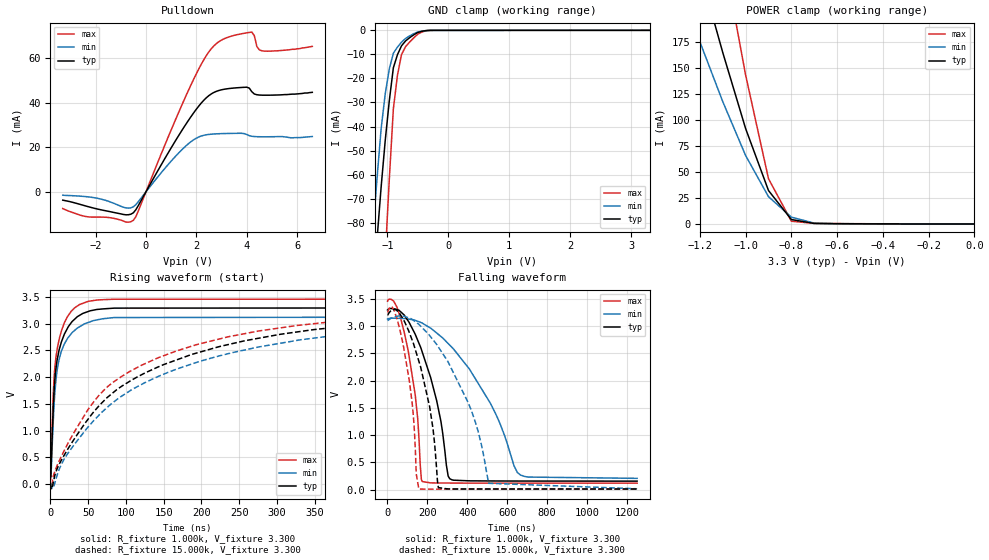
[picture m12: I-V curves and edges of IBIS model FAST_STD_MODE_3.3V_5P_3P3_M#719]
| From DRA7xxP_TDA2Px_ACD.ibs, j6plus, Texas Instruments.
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| Model based on original model for BI2C1833DVFZP18_SSCEV
|   Sub model FAST_STD_MODE_3.3V_5P_3P3
[model]   FAST_STD_MODE_3.3V_5P_3P3_M#719
|[Description]  [3.3V-I/O_OPEN_DRAIN-X-FAST MODE AND STD MODE, IND, 5 PERCENT%]
|   FAST MODE AND STD MODE, ,IND,5 PERCENT%
|[Input Load]
|[Output Drive] FAST MODE AND STD MODE
|Voltage   3.3V
|Mode   I/O_OPEN_DRAIN
Model_type   I/O_open_drain
Polarity   Non-Inverting
Enable   Active-Low
Vinl =  0.99
Vinh =  2.31
Cref =  15pF
Rref =  1000
Vref =  3.3V
Vmeas =  1.65
C_comp   2.155p   1.84p   2.47p
[Model Spec]
Vinl   0.99   0.9405   1.0395
Vinh   2.31   2.1945   2.4255
[Temperature Range]   25   125   -40
[Voltage Range]   3.3   3.135   3.465
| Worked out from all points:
|   slope of the pulldown table from 0 to 0.495 V, typ, clamps not added: 49.9 ohm
|   GND clamp passes 1 mA (typ) near -0.51 V on its own axis
|   POWER clamp passes 1 mA (typ) near -0.71 V on its own axis
|   rising waveform, R_fixture 1.000k, V_fixture 3.300: 20-80 % time 12.7ns typ, 13.7ns min, 11.4ns max; typ from 0.154 V to 3.3 V
|   rising waveform, R_fixture 15.000k, V_fixture 3.300: 20-80 % time 199ns typ, 223ns min, 173ns max; typ from 0.011 V to 3.2 V
|   falling waveform, R_fixture 1.000k, V_fixture 3.300: 20-80 % time 125ns typ, 266ns min, 69.9ns max; typ from 3.3 V to 0.155 V
|   falling waveform, R_fixture 15.000k, V_fixture 3.300: 20-80 % time 101ns typ, 203ns min, 58.8ns max; typ from 3.2 V to 0.011 V
[POWER_clamp]
-3.3V     2.049A     1.823A     3.216A
-1.233V   270.7mA    195.6mA    431mA
-1.2V     243.7mA    175.4mA    388.1mA
-1.133V   191.3mA    137mA      304.3mA
-1.1V     165.1mA    117.8mA    262.4mA
-1.067V   140.7mA    100.5mA    222.7mA
-1.033V   116.2mA    83.19mA    183mA
-1V       91.83mA    65.88mA    143.4mA
-900mV    32.17mA    26.27mA    43.57mA
-800mV    4.26mA     6.555mA    2.616mA
-700mV    450.3uA    792.4uA    566.1uA
0V        3.221uA    1.951uA    7.219uA
[Pulldown]
-3.3V     -3.73mA    -1.5mA     -7.5mA
-2.4V     -6.31mA    -2.13mA    -11.03mA
-500mV    -9.392mA   -6.725mA   -12.76mA
1.7V      32.26mA    21.71mA    45.83mA
2.4V      42.22mA    25.58mA    61.15mA
2.9V      45.45mA    26.05mA    67.36mA
4V        46.9mA     25.71mA    71.27mA
4.2V      44.88mA    24.91mA    71.61mA
4.3V      43.87mA    24.79mA    70.02mA
4.4V      43.53mA    24.72mA    65.13mA
4.6V      43.34mA    24.68mA    63.22mA
6.6V      44.6mA     24.8mA     65.2mA
[GND_clamp]
-3.3V     -875.5mA   -1.089A    -1.476A
-1.233V   -108.7mA   -83.07mA   -205.1mA
-1.167V   -86.55mA   -61.14mA   -167mA
-1.1V     -65.01mA   -40.77mA   -129.4mA
-1.033V   -45.78mA   -26.43mA   -94.2mA
-966.7mV  -29.29mA   -16.01mA   -61.94mA
-900mV    -15.55mA   -9.513mA   -32.65mA
-833.3mV  -10.16mA   -6.964mA   -18.71mA
-766.7mV  -6.44mA    -4.915mA   -10.09mA
-566.7mV  -1.886mA   -1.407mA   -3.134mA
-300mV    -12.33uA   -22.09uA   -20.16uA
3.3V      3.221uA    2.082uA    7.146uA
[Ramp]
dV/dt_f   0.966/0.26469084u   0.7119/0.70168847u   1.20204/0.13750651u
dV/dt_r   26.8524m/2.6707975n  17.96538m/4.6745527n   30.3696m/1.8597729n
R_load = 50
[Rising Waveform]
R_fixture = 1.000k
V_fixture = 3.300
V_fixture_min = 3.135
V_fixture_max = 3.465
0s        154.2mV    202.3mV    117.8mV
428.9ps   129.4mV    198mV      99.25mV
1.421ns   445.9mV    299.5mV    571.5mV
3.816ns   1.366V     1.135V     1.642V
4.812ns   1.68V      1.43V      1.936V
7.212ns   2.125V     1.897V     2.333V
9.786ns   2.371V     2.185V     2.575V
22.73ns   2.912V     2.721V     3.129V
50.42ns   3.227V     3.022V     3.416V
1.25us    3.297V     3.133V     3.458V
[Rising Waveform]
R_fixture = 15.000k
V_fixture = 3.300
V_fixture_min = 3.135
V_fixture_max = 3.465
16.52ps   10.68mV    13.73mV    7.929mV
1.137ns   -73.67mV   -28.28mV   -78.3mV
3.518ns   1.219mV    -73.46mV   110.4mV
18.14ns   537mV      465.5mV    620.9mV
49.77ns   1.211V     1.065V     1.392V
83.48ns   1.715V     1.531V     1.909V
159.6ns   2.284V     2.11V      2.452V
275.2ns   2.725V     2.562V     2.861V
550.3ns   3.098V     2.971V     3.176V
1.25us    3.204V     3.101V     3.252V
[Falling Waveform]
R_fixture = 1.000k
V_fixture = 3.300
V_fixture_min = 3.135
V_fixture_max = 3.465
577.1ps   3.297V     3.134V     3.459V
46.81ns   3.306V     3.146V     3.357V
105ns     3.091V     3.132V     2.53V
139.2ns   2.851V     3.108V     1.737V
174.4ns   2.525V     3.058V     147.4mV
246.4ns   1.635V     2.876V     121.4mV
312ns     199.4mV    2.653V     120mV
515.1ns   158.3mV    1.587V     118.1mV
666ns     156.7mV    267.5mV    117.8mV
1.25us    155.1mV    206.2mV    117.6mV
[Falling Waveform]
R_fixture = 15.000k
V_fixture = 3.300
V_fixture_min = 3.135
V_fixture_max = 3.465
589.3ps   3.204V     3.107V     3.252V
78.77ns   3.128V     3.187V     2.664V
123.8ns   2.745V     3.125V     1.589V
144.3ns   2.514V     3.07V      286.7mV
157.2ns   2.359V     3.036V     11.95mV
211.5ns   1.519V     2.828V     8.136mV
255.1ns   36.44mV    2.619V     8.029mV
424.5ns   10.72mV    1.407V     7.782mV
506.4ns   10.62mV    115.6mV    7.766mV
1.25us    10.68mV    14.75mV    7.929mV
